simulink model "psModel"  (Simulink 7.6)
settings: Solver=ode45  StartTime=psSimStruct.psSimPar.tStart  StopTime=psSimStruct.psSimPar.tStop  MaxStep=psSimStruct.psSimPar.maxStep  RelTol=psSimStruct.psSimPar.relTol
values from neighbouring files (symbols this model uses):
  psSimStruct = []    [psStartUp.m]
undefined symbols (not defined in the file or in its folder): Restriction
libraries: psModelLibrary x12

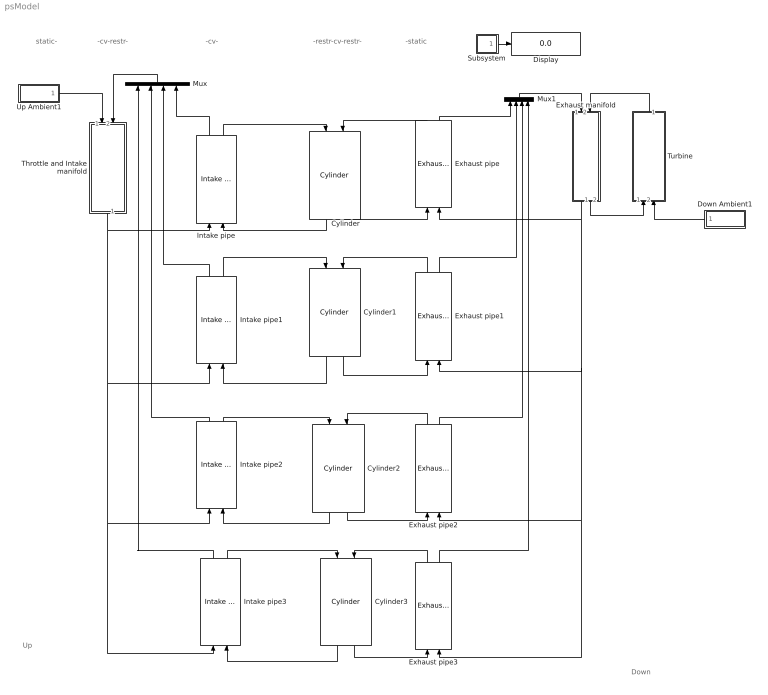
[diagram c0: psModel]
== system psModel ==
  note: -restr-cv-restr-
  note: -static
  note: Down
  note: Up
  note: static-
  note: -cv-restr-
  note: -cv-
  Cylinder : psModelLibrary/Cylinder  SystemSampleTime=-1  thetaOffset=0  CylNbr=1
  Cylinder1 : psModelLibrary/Cylinder  SystemSampleTime=-1  thetaOffset=pi  CylNbr=2
  Cylinder2 : psModelLibrary/Cylinder  SystemSampleTime=-1  thetaOffset=2*pi  CylNbr=3
  Cylinder3 : psModelLibrary/Cylinder  SystemSampleTime=-1  thetaOffset=3*pi  CylNbr=4
  Display : Display
  Down Ambient1 : Subsystem
  Exhaust manifold : Subsystem  mask{NumCyls=4}
      mask prompts: NumCyls "Number of Cylinders"
  Exhaust pipe : psModelLibrary/Exhaust pipe  SystemSampleTime=-1  CylNbr=1
  Exhaust pipe1 : psModelLibrary/Exhaust pipe  SystemSampleTime=-1  CylNbr=2
  Exhaust pipe2 : psModelLibrary/Exhaust pipe  SystemSampleTime=-1  CylNbr=3
  Exhaust pipe3 : psModelLibrary/Exhaust pipe  SystemSampleTime=-1  CylNbr=4
  Intake pipe : psModelLibrary/Intake pipe  SystemSampleTime=-1  CylNbr=1
  Intake pipe1 : psModelLibrary/Intake pipe  SystemSampleTime=-1  CylNbr=2
  Intake pipe2 : psModelLibrary/Intake pipe  SystemSampleTime=-1  CylNbr=3
  Intake pipe3 : psModelLibrary/Intake pipe  SystemSampleTime=-1  CylNbr=4
  Mux : Mux
  Mux1 : Mux
  Subsystem : Subsystem
  Throttle and Intake manifold : Subsystem  mask{NumCyls=4}
      mask prompts: NumCyls "Number of Cylinders"
  Turbine : Subsystem
  Up Ambient1 : Subsystem
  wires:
  Cylinder/2 -> Exhaust pipe/1
  Up Ambient1/1(out down) -> Throttle and Intake manifold/1(in up)
  Throttle and Intake manifold/1(out down) -> Intake pipe2/1, Intake pipe3/1, Intake pipe1/1, Intake pipe/1
  Cylinder/1 -> Intake pipe/2
  Intake pipe/2 -> Cylinder/1
  Subsystem/1(Out1) -> Display/1
  Intake pipe1/1 -> Mux/3
  Intake pipe2/1 -> Mux/2
  Intake pipe3/1 -> Mux/1
  Cylinder1/1 -> Intake pipe1/2
  Intake pipe1/2 -> Cylinder1/1
  Cylinder3/1 -> Intake pipe3/2
  Intake pipe3/2 -> Cylinder3/1
  Mux/1 -> Throttle and Intake manifold/2(in down)
  Intake pipe/1 -> Mux/4
  Cylinder1/2 -> Exhaust pipe1/1
  Cylinder2/2 -> Exhaust pipe2/1
  Cylinder3/2 -> Exhaust pipe3/1
  Intake pipe2/2 -> Cylinder2/1
  Cylinder2/1 -> Intake pipe2/2
  Exhaust pipe/1 -> Cylinder/2
  Exhaust manifold/1(out up) -> Exhaust pipe/2, Exhaust pipe1/2, Exhaust pipe2/2, Exhaust pipe3/2
  Mux1/1 -> Exhaust manifold/1(in up)
  Exhaust pipe/2 -> Mux1/1
  Exhaust manifold/2(out down) -> Turbine/1(in up)
  Down Ambient1/1(out up) -> Turbine/2(in down)
  Turbine/1(out up) -> Exhaust manifold/2(in down)
  Exhaust pipe2/1 -> Cylinder2/2
  Exhaust pipe3/1 -> Cylinder3/2
  Exhaust pipe1/1 -> Cylinder1/2
  Exhaust pipe1/2 -> Mux1/2
  Exhaust pipe2/2 -> Mux1/3
  Exhaust pipe3/2 -> Mux1/4

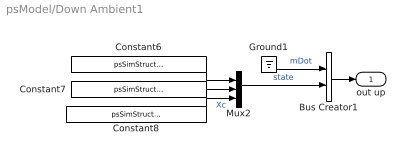
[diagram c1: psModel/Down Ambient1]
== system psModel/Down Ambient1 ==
  Bus Creator1 : BusCreator  Inputs=2
  Constant6 : Constant  Value=psSimStruct.psModel.pExh
  Constant7 : Constant  Value=psSimStruct.psModel.TExh
  Constant8 : Constant  Value=psSimStruct.psModel.XgcExh
  Ground1 : Ground
  Mux2 : Mux  Inputs=3
  out up : Outport
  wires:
  Ground1/1 -> Bus Creator1/1  "mDot"
  Mux2/1 -> Bus Creator1/2  "state"
  Constant7/1 -> Mux2/2
  Constant8/1 -> Mux2/3  "Xc"
  Bus Creator1/1 -> out up/1
  Constant6/1 -> Mux2/1

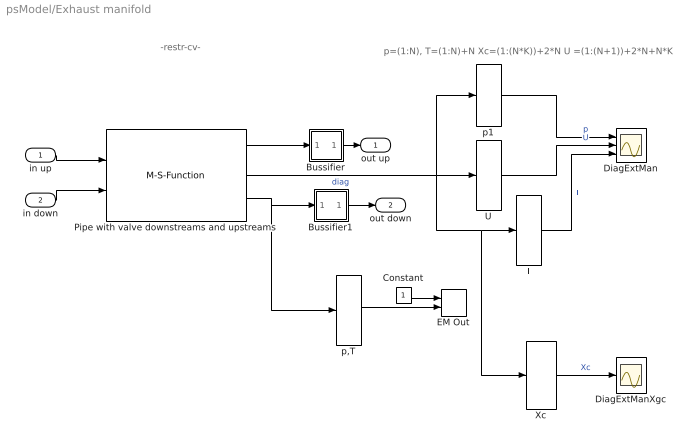
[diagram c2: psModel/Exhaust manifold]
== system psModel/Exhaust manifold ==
  note: -restr-cv-
  note: p=(1:N), T=(1:N)+N Xc=(1:(N*K))+2*N U =(1:(N+1))+2*N+N*K
  in up : Inport
  in down : Inport  Port=2
  Bussifier : Subsystem
  Bussifier1 : Subsystem
  Constant : Constant
  DiagExtMan : Scope  NumInputPorts=3
  DiagExtManXgc : Scope
  EM Out : M-S-Function  FunctionName=psToWorkspace  Parameters=2,int16('pEM TEM'),1
  Pipe with valve downstreams and upstreams : M-S-Function  FunctionName=psMultiGasPipe  Parameters=N,NumInputs,x,A,Pinit,Tinit,propInit,kFric,connectorUp,connectorDown  mask{N=1, NumInputs=[NumCyls,1], x=psSimStruct.psModel.length_common_EM, A=psSimStruct.psModel.area_common_EM, Pinit=psSimStruct.psModel.pIC_EM, Tinit=psSimStruct.psModel.TIC_EM, propInit=psSimStruct.psModel.XgcIC_EM, kFric=psSimStruct.psModel.friction_EM, connectorUp=Restriction, connectorDown=Restriction}
      mask prompts: N "Number of elements"; NumInputs "Number of inputs"; x "Pipe length [m]"; A "Pipe Area [m2]"; Pinit "Initial Pressure [Pa]"; Tinit "Initial Temperature [K]"; propInit "Initial prop [-]"; kFric "Pipe Friction"; connectorUp "Upstreams connector"; connectorDown "Downstreams connector"
  T : Selector  IndexOptions=Index vector (dialog)  Indices=(1:1)+1  OutputSizes=[(-2)]
  U : Selector  IndexOptions=Index vector (dialog)  Indices=(1:2)+2+psSimStruct.psThermProp.K  OutputSizes=[(-2)]
  Xc : Selector  IndexOptions=Index vector (dialog)  Indices=(1:(1*psSimStruct.psThermProp.K))+2*1  OutputSizes=[(-2)]
  p,T : Selector  IndexOptions=Index vector (dialog)  Indices=[2 3]  OutputSizes=[(-2)]
  p1 : Selector  IndexOptions=Index vector (dialog)  Indices=1:1  OutputSizes=[(-2)]
  out up : Outport
  out down : Outport  Port=2
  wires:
  p,T/1 -> EM Out/2
  Constant/1 -> EM Out/1
  Bussifier1/1(Out1) -> out down/1
  Pipe with valve downstreams and upstreams/1 -> Bussifier/1(In1)
  Bussifier/1(Out1) -> out up/1
  in down/1 -> Pipe with valve downstreams and upstreams/2
  in up/1 -> Pipe with valve downstreams and upstreams/1
  Pipe with valve downstreams and upstreams/3 -> p,T/1, Bussifier1/1(In1)
  U/1 -> DiagExtMan/2  "U"
  p1/1 -> DiagExtMan/1  "p"
  T/1 -> DiagExtMan/3  "T"
  Pipe with valve downstreams and upstreams/2 -> U/1, p1/1, T/1, Xc/1  "diag"
  Xc/1 -> DiagExtManXgc/1  "Xc"

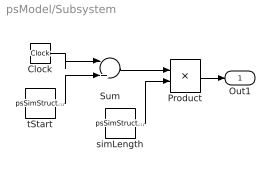
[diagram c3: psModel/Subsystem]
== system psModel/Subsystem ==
  Clock : Clock
  Product : Product  Inputs=*/
  Sum : Sum  Inputs=|+-
  simLength : Constant  Value=psSimStruct.psSimPar.tStop-psSimStruct.psSimPar.tStart
  tStart : Constant  Value=psSimStruct.psSimPar.tStart
  Out1 : Outport
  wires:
  tStart/1 -> Sum/2
  Sum/1 -> Product/1
  simLength/1 -> Product/2
  Clock/1 -> Sum/1
  Product/1 -> Out1/1

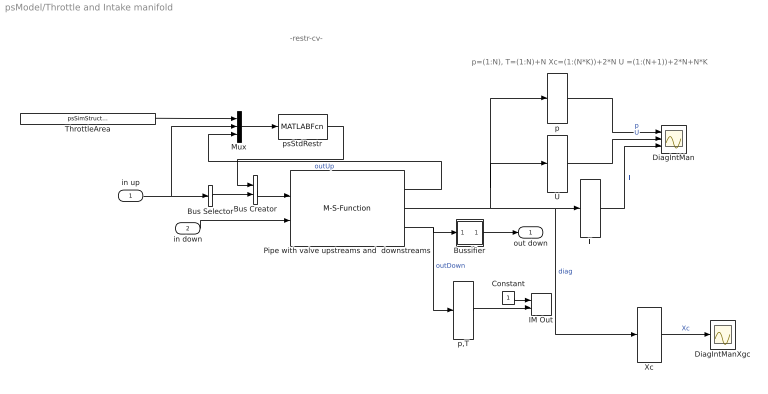
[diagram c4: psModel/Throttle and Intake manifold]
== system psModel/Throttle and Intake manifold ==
  note: -restr-cv-
  note: p=(1:N), T=(1:N)+N Xc=(1:(N*K))+2*N U =(1:(N+1))+2*N+N*K
  in up : Inport
  in down : Inport  Port=2
  Bus Creator : BusCreator  Inputs=2
  Bus Selector : BusSelector  OutputSignals=state  OutputAsBus=on
  Bussifier : Subsystem
  Constant : Constant
  DiagIntMan : Scope  NumInputPorts=3
  DiagIntManXgc : Scope
  IM Out : M-S-Function  FunctionName=psToWorkspace  Parameters=2,int16('pIM TIM'),1
  Mux : Mux  Inputs=3
  Pipe with valve upstreams and  downstreams : M-S-Function  FunctionName=psMultiGasPipe  Parameters=N,NumInputs,x,A,Pinit,Tinit,propInit,kFric,connectorUp,connectorDown  mask{N=1, NumInputs=[1,NumCyls], x=psSimStruct.psModel.length_common_IM, A=psSimStruct.psModel.area_common_IM, Pinit=psSimStruct.psModel.pIC_IM, Tinit=psSimStruct.psModel.TIC_IM, propInit=psSimStruct.psModel.XgcIC_IM, kFric=psSimStruct.psModel.friction_IM, connectorUp=Restriction, connectorDown=Restriction}
      mask prompts: N "Number of elements"; NumInputs "Number of Inputs"; x "Pipe length [m]"; A "Pipe Area [m2]"; Pinit "Initial Pressure [Pa]"; Tinit "Initial Temperature [K]"; propInit "Initial prop [-]"; kFric "Pipe Friction"; connectorUp "Upstreams connector"; connectorDown "Downstreams connector"
  T : Selector  IndexOptions=Index vector (dialog)  Indices=(1:1)+1  OutputSizes=[(-2)]
  ThrottleArea : Constant  Value=psSimStruct.psModel.ThrottleArea
  U : Selector  IndexOptions=Index vector (dialog)  Indices=(1:2)+2+psSimStruct.psThermProp.K  OutputSizes=[(-2)]
  Xc : Selector  IndexOptions=Index vector (dialog)  Indices=(1:(1*psSimStruct.psThermProp.K))+2*1  OutputSizes=[(-2)]
  p : Selector  IndexOptions=Index vector (dialog)  Indices=1  OutputSizes=[(-2)]
  p,T : Selector  IndexOptions=Index vector (dialog)  Indices=[2 3]  OutputSizes=[(-2)]
  psStdRestr : MATLABFcn  MATLABFcn=psStdRestr  OutputDimensions=1  OutputSignalType=real
  out down : Outport
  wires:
  p,T/1 -> IM Out/2
  Constant/1 -> IM Out/1
  Bussifier/1(Out1) -> out down/1
  Bus Selector/1 -> Bus Creator/2
  psStdRestr/1 -> Bus Creator/1
  Bus Creator/1 -> Pipe with valve upstreams and  downstreams/1
  Pipe with valve upstreams and  downstreams/1 -> Mux/3  "outUp"
  ThrottleArea/1 -> Mux/1
  in down/1 -> Pipe with valve upstreams and  downstreams/2
  Mux/1 -> psStdRestr/1
  in up/1 -> Bus Selector/1, Mux/2
  Pipe with valve upstreams and  downstreams/3 -> Bussifier/1(In1), p,T/1  "outDown"
  Pipe with valve upstreams and  downstreams/2 -> p/1, U/1, T/1, Xc/1  "diag"
  U/1 -> DiagIntMan/2  "U"
  p/1 -> DiagIntMan/1  "p"
  T/1 -> DiagIntMan/3  "T"
  Xc/1 -> DiagIntManXgc/1  "Xc"

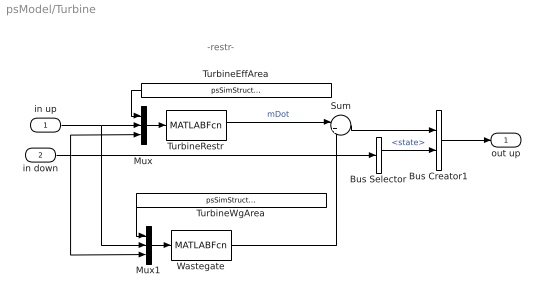
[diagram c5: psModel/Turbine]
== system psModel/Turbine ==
  note: -restr-
  in up : Inport
  in down : Inport  Port=2
  Bus Creator1 : BusCreator  Inputs=2
  Bus Selector : BusSelector  OutputSignals=state
  Mux : Mux  Inputs=3
  Mux1 : Mux  Inputs=3
  Sum : Sum  Inputs=|++
  TurbineEffArea : Constant  Value=psSimStruct.psModel.TurbineEffArea
  TurbineRestr : MATLABFcn  MATLABFcn=psTurbineRestr  OutputDimensions=1  OutputSignalType=real
  TurbineWgArea : Constant  Value=psSimStruct.psModel.TurbineWgArea
  Wastegate : MATLABFcn  MATLABFcn=psStdRestr  OutputDimensions=1  OutputSignalType=real
  out up : Outport
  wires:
  Sum/1 -> Bus Creator1/1
  Wastegate/1 -> Sum/2
  Bus Selector/1 -> Bus Creator1/2  "<state>"
  Bus Creator1/1 -> out up/1
  TurbineWgArea/1 -> Mux1/1
  Mux1/1 -> Wastegate/1
  TurbineEffArea/1 -> Mux/1
  TurbineRestr/1 -> Sum/1  "mDot"
  in down/1 -> Mux1/3, Bus Selector/1, Mux/3
  Mux/1 -> TurbineRestr/1
  in up/1 -> Mux1/2, Mux/2

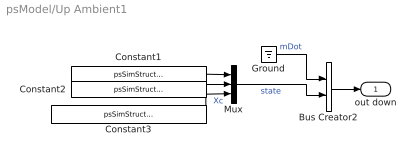
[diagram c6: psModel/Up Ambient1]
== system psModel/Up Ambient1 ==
  Bus Creator2 : BusCreator  Inputs=2
  Constant1 : Constant  Value=psSimStruct.psModel.pAmb
  Constant2 : Constant  Value=psSimStruct.psModel.TAmb
  Constant3 : Constant  Value=psSimStruct.psModel.XgcAmb
  Ground : Ground
  Mux : Mux  Inputs=3
  out down : Outport
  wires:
  Bus Creator2/1 -> out down/1
  Ground/1 -> Bus Creator2/1  "mDot"
  Mux/1 -> Bus Creator2/2  "state"
  Constant1/1 -> Mux/1
  Constant2/1 -> Mux/2
  Constant3/1 -> Mux/3  "Xc"

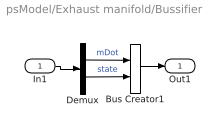
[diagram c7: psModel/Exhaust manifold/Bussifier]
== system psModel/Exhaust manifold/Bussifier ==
  In1 : Inport
  Bus Creator1 : BusCreator  Inputs=2
  Demux : Demux  Outputs=[1 2+psSimStruct.psThermProp.K]
  Out1 : Outport
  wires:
  Bus Creator1/1 -> Out1/1
  In1/1 -> Demux/1
  Demux/2 -> Bus Creator1/2  "state"
  Demux/1 -> Bus Creator1/1  "mDot"

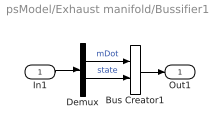
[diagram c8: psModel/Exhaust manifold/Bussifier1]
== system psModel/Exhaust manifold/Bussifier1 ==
  In1 : Inport
  Bus Creator1 : BusCreator  Inputs=2
  Demux : Demux  Outputs=[1 2+psSimStruct.psThermProp.K]
  Out1 : Outport
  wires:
  Demux/1 -> Bus Creator1/1  "mDot"
  Demux/2 -> Bus Creator1/2  "state"
  Bus Creator1/1 -> Out1/1
  In1/1 -> Demux/1

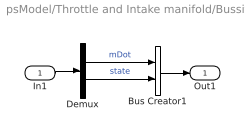
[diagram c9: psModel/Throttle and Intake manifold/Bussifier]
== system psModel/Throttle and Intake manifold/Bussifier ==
  In1 : Inport
  Bus Creator1 : BusCreator  Inputs=2
  Demux : Demux  Outputs=[1 2+psSimStruct.psThermProp.K]
  Out1 : Outport
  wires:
  In1/1 -> Demux/1
  Bus Creator1/1 -> Out1/1
  Demux/2 -> Bus Creator1/2  "state"
  Demux/1 -> Bus Creator1/1  "mDot"
